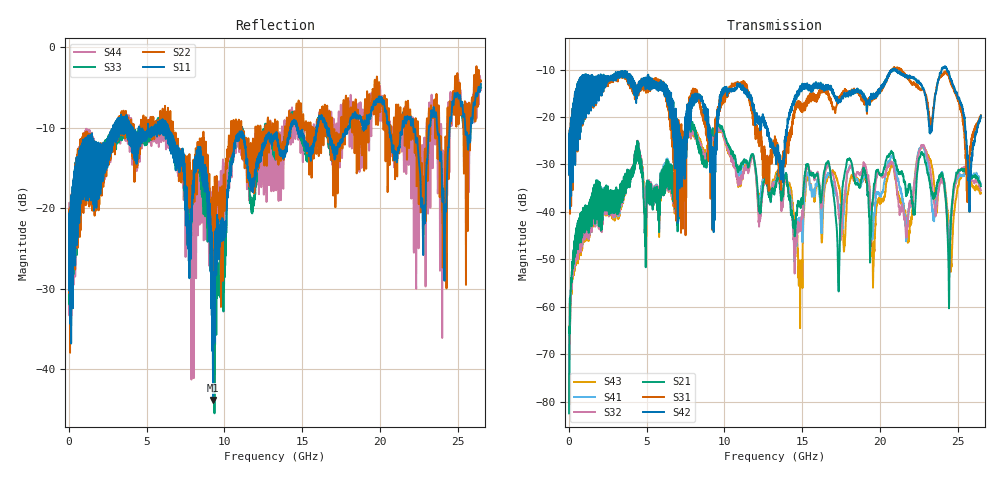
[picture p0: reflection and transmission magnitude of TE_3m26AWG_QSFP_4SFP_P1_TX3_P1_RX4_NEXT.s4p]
!Agilent Technologies,N5222A,MY51421691,A.10.00.00
!Agilent N5222A: A.10.00.00
!Date: Friday, January 30, 2015 12:34:56
!Correction: S11(Full 4 Port(1,2,3,4))
!S12(Full 4 Port(1,2,3,4))
!S13(Full 4 Port(1,2,3,4))
!S14(Full 4 Port(1,2,3,4))
!S21(Full 4 Port(1,2,3,4))
!S22(Full 4 Port(1,2,3,4))
!S23(Full 4 Port(1,2,3,4))
!S24(Full 4 Port(1,2,3,4))
!S31(Full 4 Port(1,2,3,4))
!S32(Full 4 Port(1,2,3,4))
!S33(Full 4 Port(1,2,3,4))
!S34(Full 4 Port(1,2,3,4))
!S41(Full 4 Port(1,2,3,4))
!S42(Full 4 Port(1,2,3,4))
!S43(Full 4 Port(1,2,3,4))
!S44(Full 4 Port(1,2,3,4))
!S4P File: Measurements: <S11,S12,S13,S14>,
!<S21,S22,S23,S24>,
!<S31,S32,S33,S34>,
!<S41,S42,S43,S44>:
# Hz S  dB  R 50.0
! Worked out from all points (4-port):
!   2650 points, 10 MHz to 26.5 GHz, reference 50 ohm
!   strongest paths, dB at 10 MHz, 6.63 GHz, 13.26 GHz, 19.88 GHz, 26.5 GHz:
!     S42: -25.1, -19.3, -26.9, -14.9, -19.7
!     S31: -25.0, -17.8, -24.7, -15.2, -19.6
!     S21: -82.5, -30.4, -34.9, -31.1, -34.6
!     S32: -80.3, -31.0, -34.5, -31.6, -35.5
!     S41: -80.6, -30.6, -33.9, -36.2, -34.1
!     S43: -75.0, -31.3, -32.8, -37.6, -36.1
!   lowest |S11| = -43.8 dB at 9.27 GHz (marker M1), VSWR 1.01, Z = 50 + j0.642 ohm
!   |S11| at or under -10 dB: start of sweep to 2.858 GHz; 6.364 GHz to 14.25 GHz (7.885 GHz wide, 76.5 % of centre); 16.59 GHz to 17.94 GHz (1.351 GHz wide, 7.82 % of centre)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
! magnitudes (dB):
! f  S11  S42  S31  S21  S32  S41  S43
! 10 MHz  -20.7  -25.1  -25.0  -82.5  -80.3  -80.6  -75.0
! 1.7 GHz  -11.7  -11.7  -12.1  -38.2  -39.4  -39.2  -39.7
! 9.27 GHz  -43.8  -32.8  -27.8  -23.1  -24.0  -24.1  -24.5
! 14.89 GHz  -10.4  -14.5  -16.9  -38.1  -42.5  -42.0  -51.4
! 15.36 GHz  -12.4  -13.4  -16.8  -30.3  -30.6  -32.2  -32.7
! 17.33 GHz  -12.0  -17.0  -16.4  -55.1  -39.2  -38.4  -34.2
! 26.5 GHz  -4.6  -19.7  -19.6  -34.6  -35.5  -34.1  -36.1
